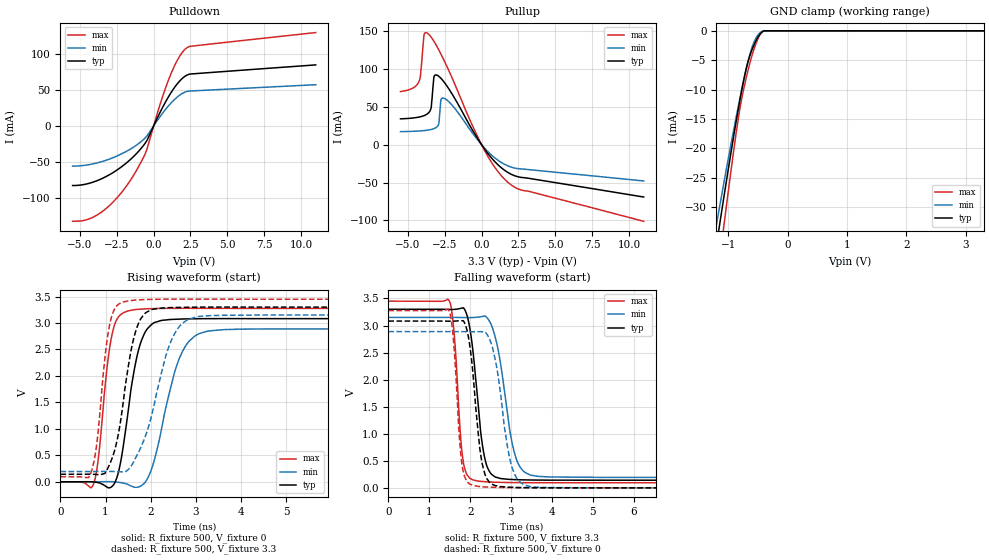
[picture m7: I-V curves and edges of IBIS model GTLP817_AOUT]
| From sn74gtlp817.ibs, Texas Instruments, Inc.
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[Model]   GTLP817_AOUT
Model_type  3-state
Enable   Active-Low
Vref =   0
Rref =   500
Cref =   50p
Vmeas =   1.5
| variable   typ   min   max
C_comp   3.04pF   2.61pF   3.72pF
| C_pullup   3.63pF   2.85pF   4.52pF
| C_pulldown   3.82pF   3.02pF   4.59pF
| C_tri-state   3.04pF   2.61pF   3.72pF
[Temperature Range]   40   100   -40
| Ambient temperature   25   85   -40
[Voltage range]   3.3   3.15   3.45
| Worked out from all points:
|   slope of the pulldown table from 0 to 0.495 V, typ, clamps not added: 23.3 ohm
|   slope of the pullup table from 0 to 0.495 V, typ, clamps not added: 37.1 ohm
|   GND clamp passes 1 mA (typ) near -0.49 V on its own axis
|   rising waveform, R_fixture 500, V_fixture 0: 20-80 % time 341ps typ, 494ps min, 240ps max; typ from 0 V to 3.08 V
|   falling waveform, R_fixture 500, V_fixture 3.3: 20-80 % time 258ps typ, 357ps min, 169ps max; typ from 3.3 V to 0.142 V
|   rising waveform, R_fixture 500, V_fixture 3.3: 20-80 % time 359ps typ, 557ps min, 240ps max; typ from 0.142 V to 3.3 V
|   falling waveform, R_fixture 500, V_fixture 0: 20-80 % time 238ps typ, 330ps min, 163ps max; typ from 3.08 V to 0 V
[GND Clamp]
| GTLP817_AOUT
|   Voltage   I(typ)   I(min)   I(max)
-5.5V     -354.5mA   -306.5mA   -437.6mA
-1.195V   -36.4mA    -32.86mA   -43.16mA
-1.145V   -33.09mA   -30.01mA   -39.08mA
-1.1V     -30.15mA   -27.46mA   -35.45mA
-1.055V   -27.23mA   -24.94mA   -31.85mA
-835mV    -13.65mA   -13.14mA   -15.3mA
-780mV    -10.56mA   -10.4mA    -11.99mA
-700mV    -6.606mA   -6.678mA   -8.169mA
-565mV    -2.394mA   -1.919mA   -3.1mA
-490mV    -932.6uA   -609.6uA   -1.16mA
-420mV    -129.2uA   -61.65uA   -133.3uA
3.3V      167pA      18.09nA    -3.027nA
[Pulldown]
| GTLP817_AOUT
|   Voltage   I(typ)   I(min)   I(max)
-5.5V     -82.89mA   -55.89mA   -132.6mA
-4.51V    -80.53mA   -54.31mA   -130.2mA
-3.555V   -73.69mA   -49.87mA   -120.1mA
-2.54V    -62.07mA   -42.31mA   -101.2mA
-1.56V    -46.39mA   -32.02mA   -75.09mA
-520mV    -22.36mA   -15.51mA   -35.89mA
505mV     21.64mA    14.91mA    34.31mA
1.21V     47.24mA    32.49mA    74.09mA
1.735V    61.68mA    42.26mA    95.87mA
2.215V    70.09mA    47.59mA    108mA
2.5V      72.13mA    48.49mA    110.7mA
11V       84.83mA    57.26mA    129.8mA
[Pullup]
| GTLP817_AOUT
|   Voltage   I(typ)   I(min)   I(max)
-5.5V     34.15mA    17.24mA    70.17mA
-4.255V   36.46mA    18.09mA    83.08mA
-3.91V    38.32mA    18.64mA    144.3mA
-3.705V   40.34mA    19.12mA    147.7mA
-3.42V    49.11mA    20.13mA    142mA
-3.225V   89.91mA    21.29mA    136.3mA
-2.935V   90.79mA    25.99mA    126.4mA
-2.76V    87.71mA    59.09mA    119.9mA
-2.465V   80.66mA    60.59mA    108.1mA
135mV     -3.881mA   -3.047mA   -5.131mA
1.78V     -36.63mA   -27.95mA   -49.59mA
11V       -69.11mA   -47.87mA   -101.2mA
[Ramp]
| GTLP817_AOUT
| variable   typ   min   max
dV/dt_r   1.92/3.61E-10   1.80/5.23E-10   2.03/2.56E-10
dV/dt_f   1.91/2.69E-10   1.79/3.71E-10   2.04/1.78E-10
R_load = 500
[Rising Waveform]
| GTLP817_AOUT
R_fixture =   500
C_fixture =   0
L_fixture =   0
V_fixture =   0
V_fixture_min = 0
V_fixture_max = 0
|   Time   V(typ)   V(min)   V(max)
0s        -4.856uV   -397.4nV   -6.605uV
740ps     -2.855mV   323.4uV    -25.97mV
1.06ns    -114.1mV   2.453mV    2.348V
1.185ns   -48.48mV   -794.7uV   2.925V
1.35ns    446mV      -16.98mV   3.168V
1.635ns   2.107V     -100.2mV   3.251V
2.015ns   2.969V     228.3mV    3.272V
2.69ns    3.075V     2.436V     3.278V
3.305ns   3.082V     2.852V     3.277V
24.99ns   3.082V     2.886V     3.276V
[Falling Waveform]
| GTLP817_AOUT
R_fixture =   500
C_fixture =   0
L_fixture =   0
V_fixture =   3.3
V_fixture_min = 3.15
V_fixture_max = 3.45
|   Time   V(typ)   V(min)   V(max)
0s        3.3V       3.15V      3.45V
1.49ns    3.297V     3.15V      3.453V
1.605ns   3.298V     3.15V      2.884V
1.835ns   3.327V     3.148V     468.8mV
2.01ns    2.864V     3.146V     168.7mV
2.19ns    1.59V      3.155V     126.5mV
2.495ns   274.6mV    3.047V     107.8mV
3.105ns   152mV      590mV      97.54mV
3.61ns    144.1mV    217.8mV    95.34mV
24.99ns   141.8mV    193.7mV    94.08mV
[Rising Waveform]
| GTLP817_AOUT
R_fixture =   500
C_fixture =   0
L_fixture =   0
V_fixture =   3.3
V_fixture_min = 3.15
V_fixture_max = 3.45
|   Time   V(typ)   V(min)   V(max)
0s        141.8mV    193.6mV    94.06mV
670ps     142.6mV    193.7mV    158.9mV
800ps     137.8mV    194.2mV    685.7mV
1.105ns   359mV      196.1mV    3.024V
1.285ns   906mV      190mV      3.353V
1.51ns    2.21V      235.3mV    3.419V
1.89ns    3.193V     876.8mV    3.444V
2.47ns    3.292V     2.694V     3.451V
3.08ns    3.3V       3.125V     3.451V
24.99ns   3.3V       3.15V      3.45V
[Falling Waveform]
| GTLP817_AOUT
R_fixture =   500
C_fixture =   0
L_fixture =   0
V_fixture =   0
V_fixture_min = 0
V_fixture_max = 0
|   Time   V(typ)   V(min)   V(max)
0s        3.082V     2.888V     3.276V
1.48ns    3.08V      2.888V     3.275V
1.59ns    3.081V     2.888V     2.749V
1.8ns     3.089V     2.886V     434.9mV
1.96ns    2.776V     2.885V     90.3mV
2.11ns    1.743V     2.886V     38.38mV
2.405ns   172.7mV    2.845V     15.09mV
3.005ns   11.03mV    428.2mV    3.882mV
3.455ns   2.977mV    26.57mV    1.593mV
24.99ns   29.99uV    93.6uV     16.36uV
